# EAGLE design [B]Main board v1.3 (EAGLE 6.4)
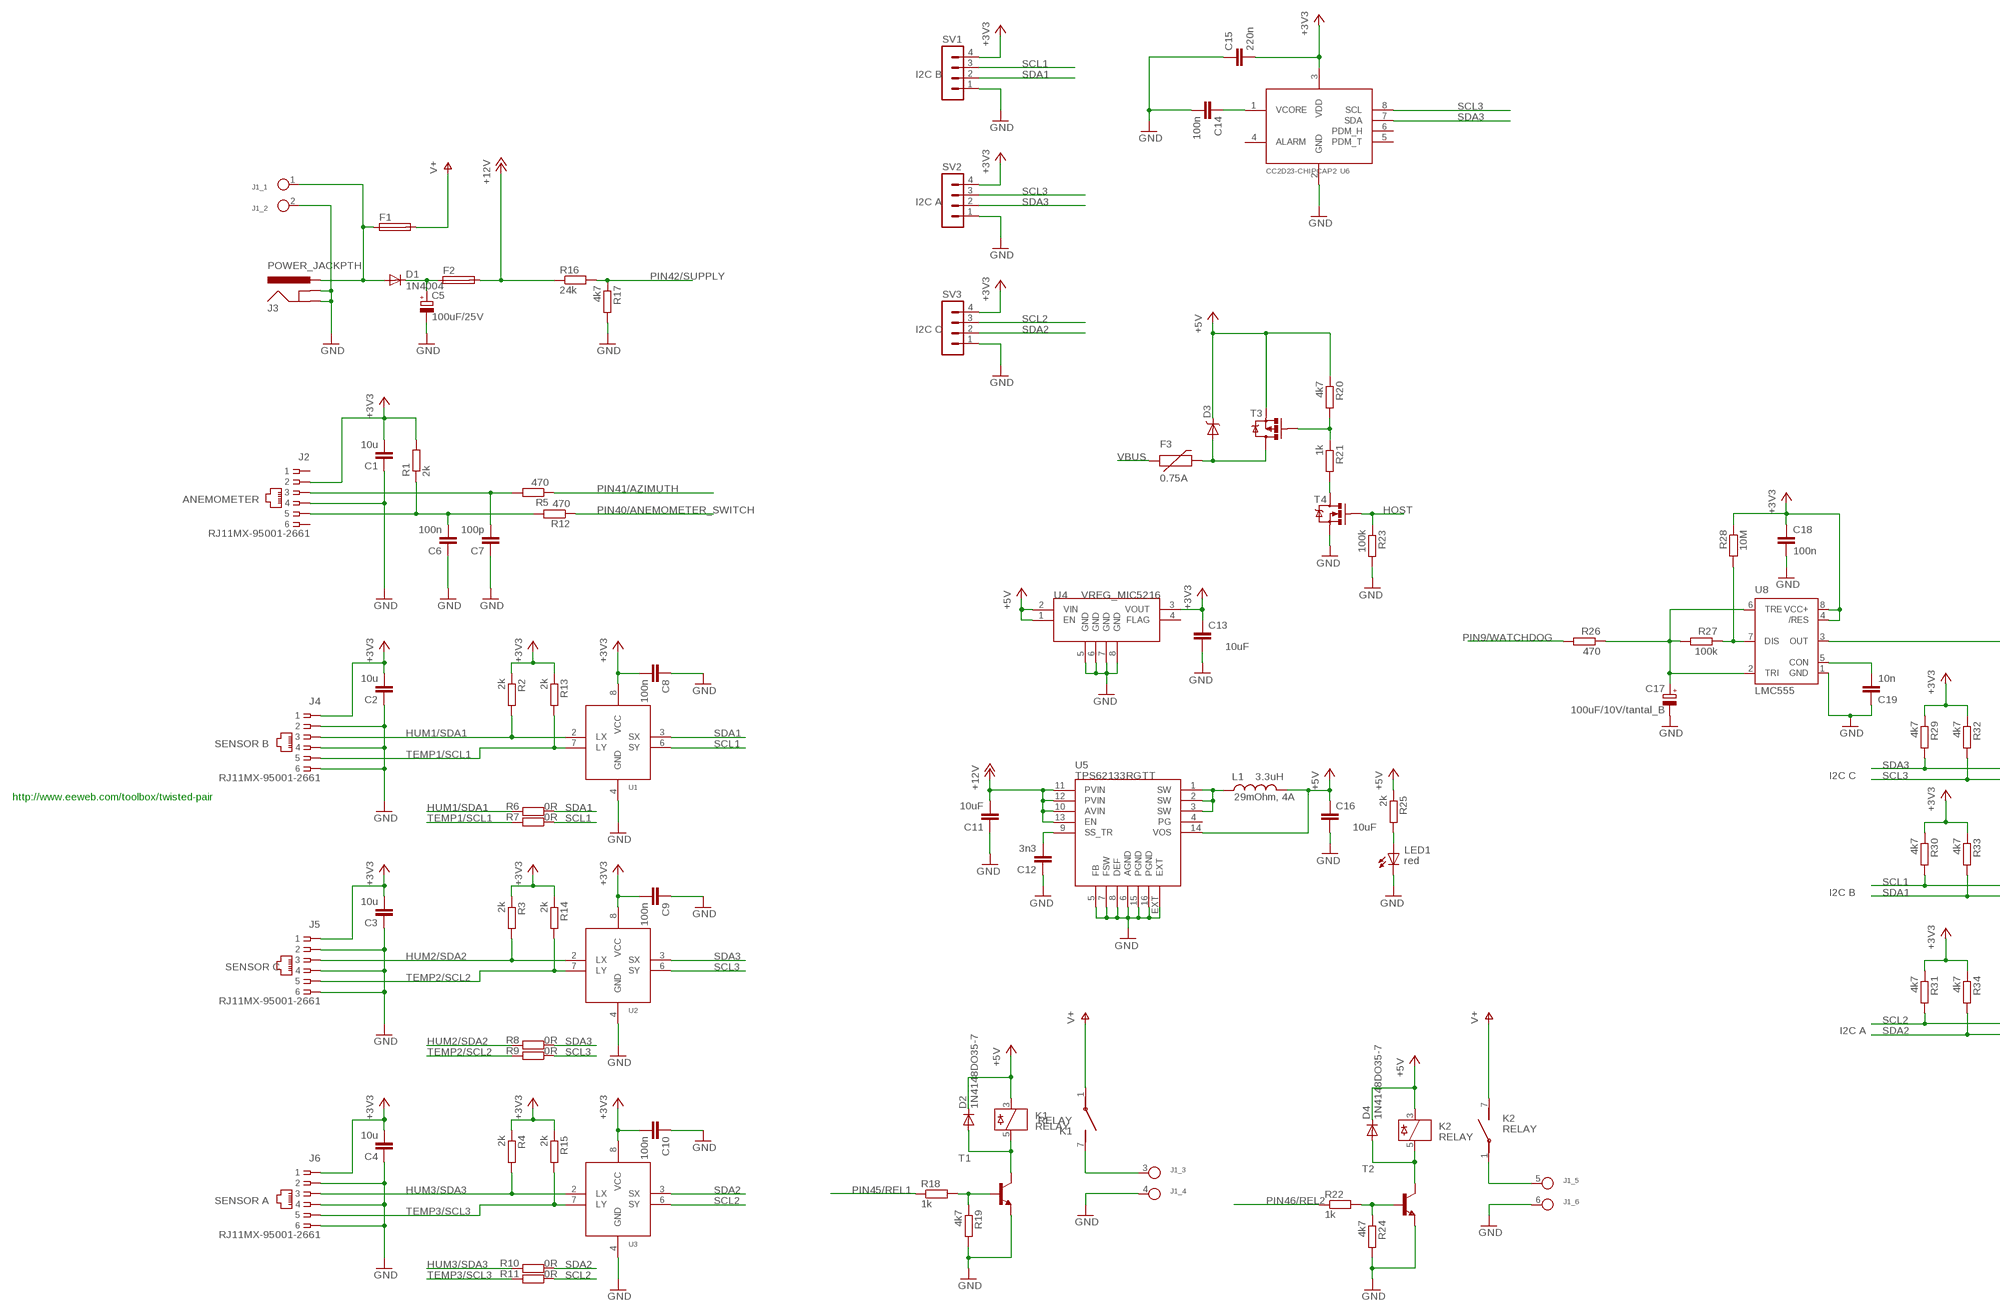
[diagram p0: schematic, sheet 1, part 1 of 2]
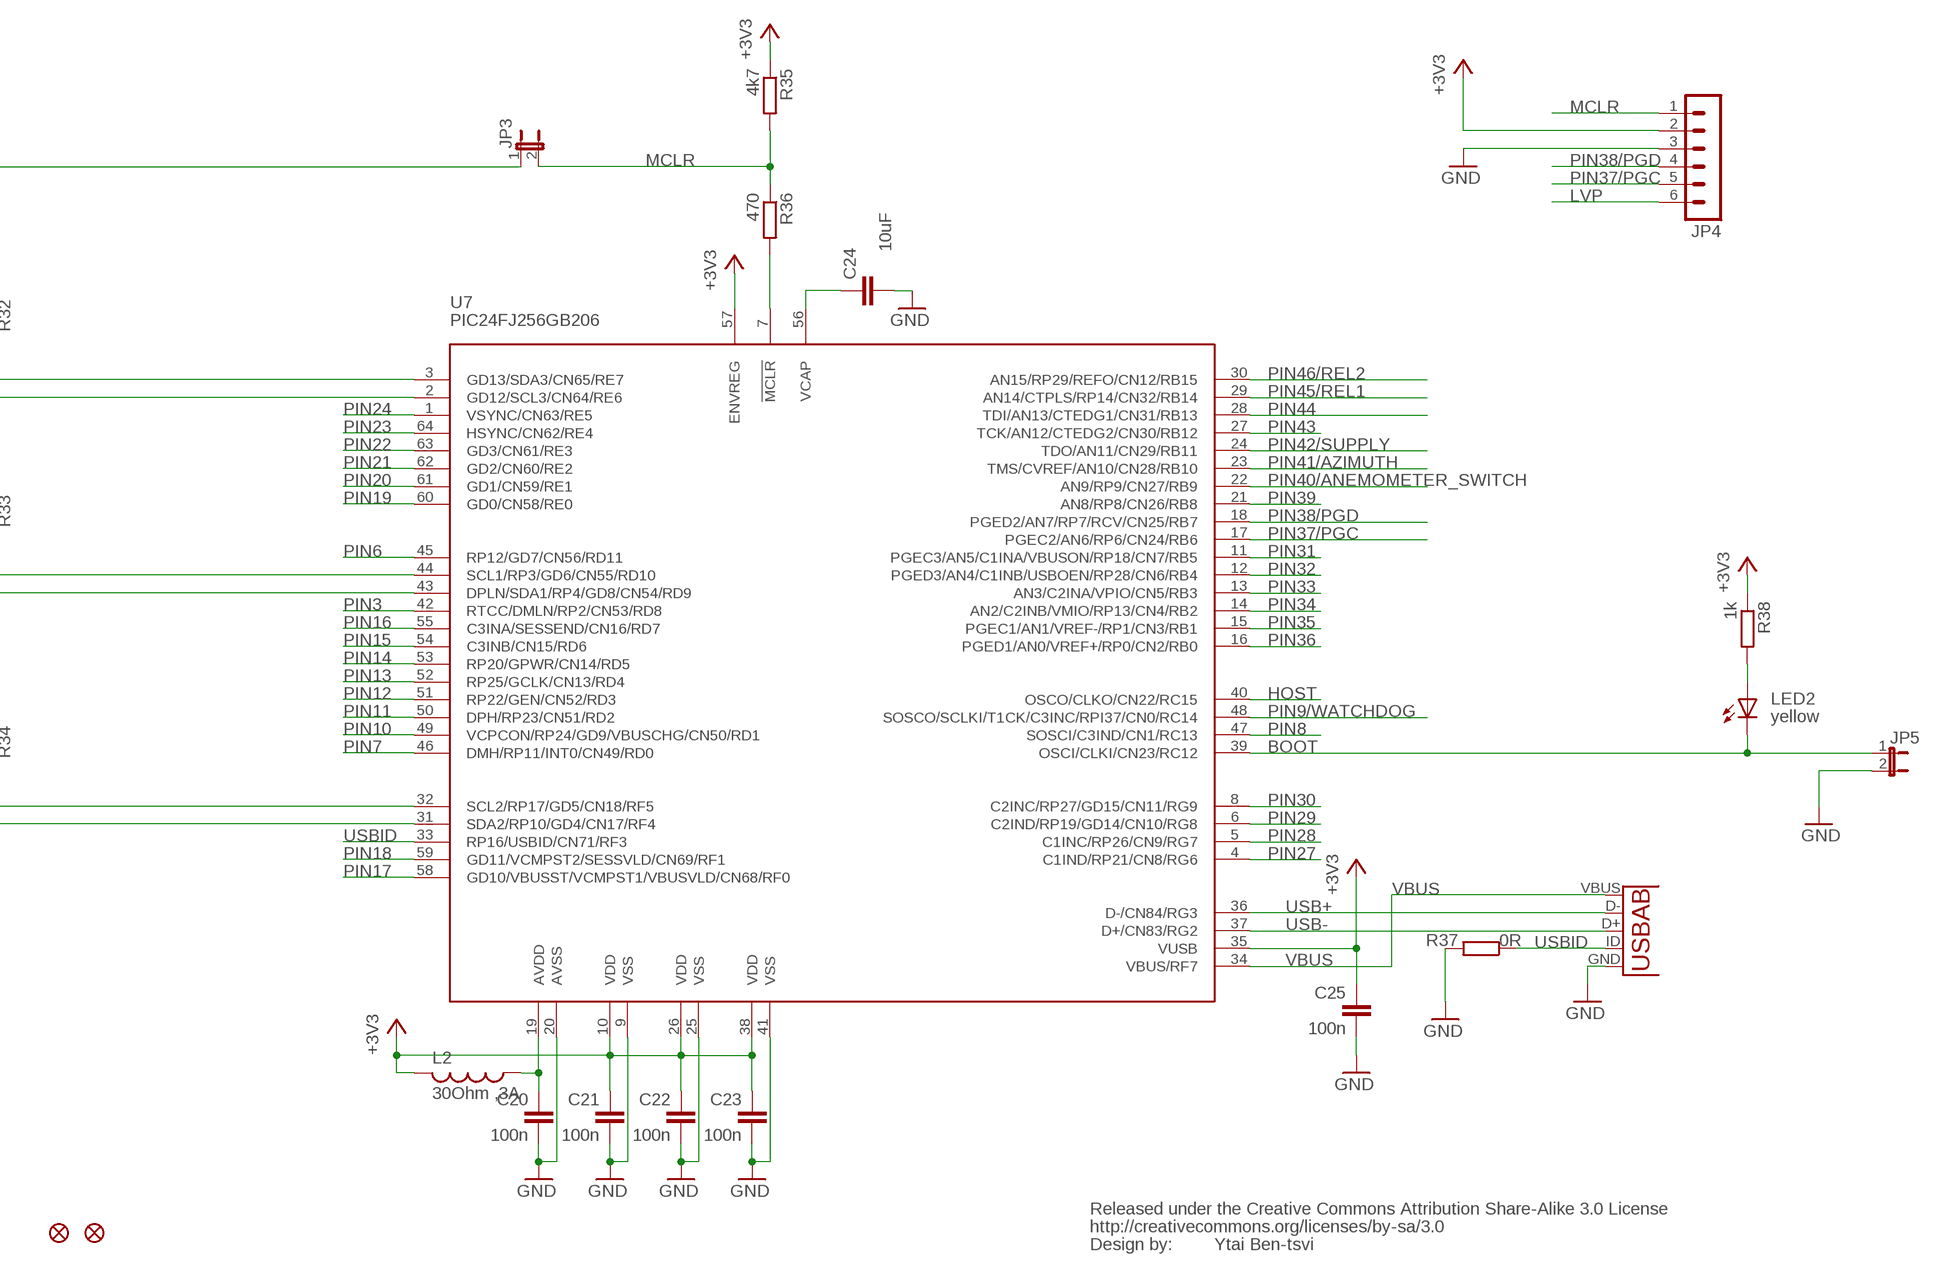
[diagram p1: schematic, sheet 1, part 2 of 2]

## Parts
C1  10u  C-EUC1206  [C1206]
C2  10u  C-EUC1206  [C1206]
C3  10u  C-EUC1206  [C1206]
C4  10u  C-EUC1206  [C1206]
C5  100uF/25V  CPOL-EUE2-5  [E2-5]
C6  100n  C-EUC1206  [C1206]
C7  100p  C-EUC1206  [C1206]
C8  100n  C-EUC1206  [C1206]
C9  100n  C-EUC1206  [C1206]
C10  100n  C-EUC1206  [C1206]
C11  10uF  C-EUC1206  [C1206]
C12  3n3  C-EUC1206  [C1206]
C13  10uF  C-EUC1206  [C1206]
C14  100n  C-EUC1206  [C1206]
C15  220n  C-EUC1206  [C1206]
C16  10uF  C-EUC1206  [C1206]
C17  100uF/10V/tantal_B  CPOL-EUB/3528-21R  [B/3528-21R]
C18  100n  C-EUC1206  [C1206]
C19  10n  C-EUC1206  [C1206]
C20  100n  C-EUC1206  [C1206]
C21  100n  C-EUC1206  [C1206]
C22  100n  C-EUC1206  [C1206]
C23  100n  C-EUC1206  [C1206]
C24  10uF  C-EUC1206  [C1206]
C25  100n  C-EUC1206  [C1206]
D1  1N4004  [DO41-10]
D2  1N4148DO35-7  [DO35-7]
D3  B340A  DIODE-SCHOTTKY_  [SMA-DIODE]
D4  1N4148DO35-7  [DO35-7]
F1  FUSE_HOLDER  [ZHL30]
F2  FUSE_HOLDER  [ZHL30]
F3  PTCSMD  [PTC-1206]
J1  6P_CONN  [MOLEX_39543-0006]
J2  RJ11MX-95001-2661  [MX-95001-2661]
J3  POWER_JACKPTH  [PC-GK2.1]
J4  RJ11MX-95001-2661  [MX-95001-2661]
J5  RJ11MX-95001-2661  [MX-95001-2661]
J6  RJ11MX-95001-2661  [MX-95001-2661]
J7  10104111-0001LF  USB_AB  [USB-AB-MICRO-SMD]
JP1  FIDUCIALUFIDUCIAL  [MICRO-FIDUCIAL]
JP2  FIDUCIALUFIDUCIAL  [MICRO-FIDUCIAL]
JP3  JUMPER-2PTH  [1X02]
JP4  MA06-1  [MA06-1]
JP5  JUMPER-2PTH  [1X02]
K1  RELAY  [JV-5S-KT]
K2  RELAY  [JV-5S-KT]
L1  VLC5045T-3R3N  INDUCTORCR54  [CR54]
L2  30Ohm ,3A  L-US  [R1206]
LED1  LS L29K-G1J2-1-Z  LED1206  [LED-1206]
LED2  LY L29K-J1K2-26-Z  LED1206  [LED-1206]
R1  2k  R-EU_R1206  [R1206]
R2  2k  R-EU_R1206  [R1206]
R3  2k  R-EU_R1206  [R1206]
R4  2k  R-EU_R1206  [R1206]
R5  470  R-EU_R1206  [R1206]
R6  0R  R-EU_R1206  [R1206]
R7  0R  R-EU_R1206  [R1206]
R8  0R  R-EU_R1206  [R1206]
R9  0R  R-EU_R1206  [R1206]
R10  0R  R-EU_R1206  [R1206]
R11  0R  R-EU_R1206  [R1206]
R12  470  R-EU_R1206  [R1206]
R13  2k  R-EU_R1206  [R1206]
R14  2k  R-EU_R1206  [R1206]
R15  2k  R-EU_R1206  [R1206]
R16  24k  R-EU_R1206  [R1206]
R17  4k7  R-EU_R1206  [R1206]
R18  1k  R-EU_R1206  [R1206]
R19  4k7  R-EU_R1206  [R1206]
R20  4k7  R-EU_R1206  [R1206]
R21  1k  R-EU_R1206  [R1206]
R22  1k  R-EU_R1206  [R1206]
R23  100k  R-EU_R1206  [R1206]
R24  4k7  R-EU_R1206  [R1206]
R25  2k  R-EU_R1206  [R1206]
R26  470  R-EU_R1206  [R1206]
R27  100k  R-EU_R1206  [R1206]
R28  10M  R-EU_R1206  [R1206]
R29  4k7  R-EU_R1206  [R1206]
R30  4k7  R-EU_R1206  [R1206]
R31  4k7  R-EU_R1206  [R1206]
R32  4k7  R-EU_R1206  [R1206]
R33  4k7  R-EU_R1206  [R1206]
R34  4k7  R-EU_R1206  [R1206]
R35  4k7  R-EU_R1206  [R1206]
R36  470  R-EU_R1206  [R1206]
R37  0R  R-EU_R1206  [R1206]
R38  1k  R-EU_R1206  [R1206]
SV1  MA04-1  [MA04-1]
SV2  MA04-1  [MA04-1]
SV3  MA04-1  [MA04-1]
T1  BC817-16-NPN-SOT23-BEC  [SOT23-BEC]
T2  BC817-16-NPN-SOT23-BEC  [SOT23-BEC]
T3  IRLML2244  MOSFET-PCHANNELSMD  [SOT23-3]
T4  2N7002PW  MOSFET-NCHANNELSOT323  [SOT323]
U1  P82B715_I2C_BUS_EXTENDER  [SO-08]
U2  P82B715_I2C_BUS_EXTENDER  [SO-08]
U3  P82B715_I2C_BUS_EXTENDER  [SO-08]
U4  VREG_MIC5216  [MSOP8]
U5  TPS62133RGTT  TPS6214X  [QFN16-3X3MM]
U6  CC2D23-CHIPCAP2  [CC2D23-CHIPCAP2]
U7  PIC24FJ256GB206  PIC24FXXXDAX06  [PIC24FXXX_TQFP64]
U8  LMC555  NE555D  [SO08]
U$1  CREATIVE_COMMONS  [CREATIVE_COMMONS]

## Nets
+3V3: C1.2 C2.2 C3.2 C4.2 C8.2 C9.2 C10.2 C13.2 C15.2 C18.1 C21.1 C22.1 C23.1 C25.1 J2.2 J4.1 J5.1 J6.1 JP4.2 L2.2 R1.2 R2.1 R3.1 R4.1 R13.1 R14.1 R15.1 R28.1 R29.1 R30.1 R31.1 R32.1 R33.1 R34.1 R35.1 R38.1 SV1.4 SV2.4 SV3.4 U1.8(VCC) U2.8(VCC) U3.8(VCC) U4.3(VOUT) U6.3(VDD) U7.10(VDD) U7.26(VDD) U7.35(VUSB) U7.38(VDD) U7.57(ENVREG) U8.4(/RES) U8.8(VCC+)
+5V [VCC]: C16.2 D2.C D3.C D4.C K1.3 K2.3 L1.P$2 R20.1 R25.1 T3.2(S) U4.1(EN) U4.2(VIN) U5.14(VOS)
+12V: C11.2 F2.2 R16.1 U5.10(AVIN) U5.11(PVIN) U5.12(PVIN) U5.13(EN)
BOOT: JP5.1 LED2.C U7.39(OSCI/CLKI/CN23/RC12)
GND [VCC]: C1.1 C2.1 C3.1 C4.1 C5.- C6.1 C7.1 C8.1 C9.1 C10.1 C11.1 C12.1 C13.1 C14.2 C15.1 C16.1 C17.- C18.2 C19.1 C20.2 C21.2 C22.2 C23.2 C24.1 C25.2 J1.2 J1.4 J1.6 J2.4 J3.GND J3.GNDBREAK J4.2 J4.4 J4.6 J5.2 J5.4 J5.6 J6.2 J6.4 J6.6 J7.GND JP4.3 JP5.2 LED1.C R17.2 R19.2 R23.2 R24.2 R37.2 SV1.1 SV2.1 SV3.1 T1.E T2.E T4.2(S) U1.4(GND) U2.4(GND) U3.4(GND) U4.5(GND) U4.6(GND) U4.7(GND) U4.8(GND) U5.5(FB) U5.6(AGND) U5.7(FSW) U5.8(DEF) U5.15(PGND) U5.16(PGND) U5.EXT U6.2(GND) U7.9(VSS) U7.20(AVSS) U7.25(VSS) U7.41(VSS) U8.1(GND)
HOST: R23.1 T4.1(G) U7.40(OSCO/CLKO/CN22/RC15)
HUM1/SDA1: J4.3 R2.2 R6.2 U1.2(LX)
HUM2/SDA2: J5.3 R3.2 R8.2 U2.2(LX)
HUM3/SDA3: J6.3 R4.2 R10.2 U3.2(LX)
LVP: JP4.6
MCLR: JP3.2 JP4.1 R35.2 R36.1
N$1: D1.A F1.1 J1.1 J3.PWR
N$2: C6.2 J2.5 R1.1 R12.2
N$3: C5.+ D1.C F2.1
N$4: C7.2 J2.3 R5.2
N$6: C14.1 U6.1(VCORE)
N$9: R36.2 U7.7(!MCLR)
N$10: JP3.1 U8.3(OUT)
N$11: R18.2 R19.1 T1.B
N$12: D2.A K1.5 T1.C
N$13: C19.2 U8.5(CON)
N$16: J1.3 K1.7(2:S)
N$17: C17.+ R26.1 R27.2 U8.2(TRI) U8.6(TRE)
N$19: R27.1 R28.2 U8.7(DIS)
N$20: R22.2 R24.1 T2.B
N$21: D4.A K2.5 T2.C
N$22: C24.2 U7.56(VCAP)
N$23: J1.5 K2.1(2:P)
N$24: LED2.A R38.2
N$25: LED1.A R25.2
N$26: D3.A F3.2 T3.3(D)
N$27: C12.2 U5.9(SS_TR)
N$28: L1.P$1 U5.1(SW) U5.2(SW) U5.3(SW)
N$29: C20.1 L2.1 U7.19(AVDD)
N$30: R20.2 R21.1 T3.1(G)
N$31: R21.2 T4.3(D)
PIN3: U7.42(RTCC/DMLN/RP2/CN53/RD8)
PIN6: U7.45(RP12/GD7/CN56/RD11)
PIN7: U7.46(DMH/RP11/INT0/CN49/RD0)
PIN8: U7.47(SOSCI/C3IND/CN1/RC13)
PIN9/WATCHDOG: R26.2 U7.48(SOSCO/SCLKI/T1CK/C3INC/RPI37/CN0/RC14)
PIN10: U7.49(VCPCON/RP24/GD9/VBUSCHG/CN50/RD1)
PIN11: U7.50(DPH/RP23/CN51/RD2)
PIN12: U7.51(RP22/GEN/CN52/RD3)
PIN13: U7.52(RP25/GCLK/CN13/RD4)
PIN14: U7.53(RP20/GPWR/CN14/RD5)
PIN15: U7.54(C3INB/CN15/RD6)
PIN16: U7.55(C3INA/SESSEND/CN16/RD7)
PIN17: U7.58(GD10/VBUSST/VCMPST1/VBUSVLD/CN68/RF0)
PIN18: U7.59(GD11/VCMPST2/SESSVLD/CN69/RF1)
PIN19: U7.60(GD0/CN58/RE0)
PIN20: U7.61(GD1/CN59/RE1)
PIN21: U7.62(GD2/CN60/RE2)
PIN22: U7.63(GD3/CN61/RE3)
PIN23: U7.64(HSYNC/CN62/RE4)
PIN24: U7.1(VSYNC/CN63/RE5)
PIN27: U7.4(C1IND/RP21/CN8/RG6)
PIN28: U7.5(C1INC/RP26/CN9/RG7)
PIN29: U7.6(C2IND/RP19/GD14/CN10/RG8)
PIN30: U7.8(C2INC/RP27/GD15/CN11/RG9)
PIN31: U7.11(PGEC3/AN5/C1INA/VBUSON/RP18/CN7/RB5)
PIN32: U7.12(PGED3/AN4/C1INB/USBOEN/RP28/CN6/RB4)
PIN33: U7.13(AN3/C2INA/VPIO/CN5/RB3)
PIN34: U7.14(AN2/C2INB/VMIO/RP13/CN4/RB2)
PIN35: U7.15(PGEC1/AN1/VREF-/RP1/CN3/RB1)
PIN36: U7.16(PGED1/AN0/VREF+/RP0/CN2/RB0)
PIN37/PGC: JP4.5 U7.17(PGEC2/AN6/RP6/CN24/RB6)
PIN38/PGD: JP4.4 U7.18(PGED2/AN7/RP7/RCV/CN25/RB7)
PIN39: U7.21(AN8/RP8/CN26/RB8)
PIN40/ANEMOMETER_SWITCH: R12.1 U7.22(AN9/RP9/CN27/RB9)
PIN41/AZIMUTH: R5.1 U7.23(TMS/CVREF/AN10/CN28/RB10)
PIN42/SUPPLY: R16.2 R17.1 U7.24(TDO/AN11/CN29/RB11)
PIN43: U7.27(TCK/AN12/CTEDG2/CN30/RB12)
PIN44: U7.28(TDI/AN13/CTEDG1/CN31/RB13)
PIN45/REL1: R18.1 U7.29(AN14/CTPLS/RP14/CN32/RB14)
PIN46/REL2: R22.1 U7.30(AN15/RP29/REFO/CN12/RB15)
SCL1: R7.1 R30.2 SV1.3 U1.6(SY) U7.44(SCL1/RP3/GD6/CN55/RD10)
SCL2: R11.1 R31.2 SV3.3 U3.6(SY) U7.32(SCL2/RP17/GD5/CN18/RF5)
SCL3: R9.1 R32.2 SV2.3 U2.6(SY) U6.8(SCL) U7.2(GD12/SCL3/CN64/RE6)
SDA1: R6.1 R33.2 SV1.2 U1.3(SX) U7.43(DPLN/SDA1/RP4/GD8/CN54/RD9)
SDA2: R10.1 R34.2 SV3.2 U3.3(SX) U7.31(SDA2/RP10/GD4/CN17/RF4)
SDA3: R8.1 R29.2 SV2.2 U2.3(SX) U6.7(SDA) U7.3(GD13/SDA3/CN65/RE7)
TEMP1/SCL1: J4.5 R7.2 R13.2 U1.7(LY)
TEMP2/SCL2: J5.5 R9.2 R14.2 U2.7(LY)
TEMP3/SCL3: J6.5 R11.2 R15.2 U3.7(LY)
USB+: J7.D- U7.36(D-/CN84/RG3)
USB-: J7.D+ U7.37(D+/CN83/RG2)
USBID: J7.ID(USBID) R37.1 U7.33(RP16/USBID/CN71/RF3)
V+: F1.2 K1.1(2:P) K2.7(2:S)
VBUS: F3.1 J7.VBUS U7.34(VBUS/RF7)
Unconnected: J2.1 J2.6 U4.4(FLAG) U5.4(PG) U6.4(ALARM) U6.5(PDM_T) U6.6(PDM_H)

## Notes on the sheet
- I2C B
- I2C A
- I2C C
- 0.75A
- ANEMOMETER
- SENSOR B
- I2C C
- http://www.eeweb.com/toolbox/twisted-pair | 29mOhm, 4A
- red
- I2C B
- SENSOR C
- yellow
- I2C A
- SENSOR A
- Ytai Ben-tsvi

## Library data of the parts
C1-C4 C6-C16 C18-C25 = rcl:C-EU: CAPACITOR, European symbol
C5 = Thomas Egnal Library:CPOL-EU: POLARIZED CAPACITOR, European symbol
C17 = rcl:CPOL-EU: POLARIZED CAPACITOR, European symbol
D1 = diode:1N4004: DIODE
D2 D4 = diode:1N4148: DIODE
D3 = SparkFun-DiscreteSemi:DIODE-SCHOTTKY: Commonly MBRA140.; PART#: B340A
F1 F2 = Thomas Egnal Library:FUSE_HOLDER: http://www.tme.eu/pl/details/zhl30/bezpieczniki-gniazda-pcb/#t735977d29e6b3d766657895563ce61ae
F3 = SparkFun-PowerIC:PTC: Resettable Fuse PTC; PART#: 0ZCA0075FF2G
J1 = Thomas Egnal Library:6P_CONN
J2 J4-J6 = Thomas Egnal Library:RJ11: CORCOM Modular RJ Jacks No Shield Source: https://www.elfa.se/elfa3~se_sv/elfa/init.do?item=42-696-27&toc=0&q=42-696-27
J3 = Thomas Egnal Library:POWER_JACK: Power Jack This is the standard 5.5mm barrel jack for power. The PTH is the most common, proven, reliable, footprint. All others are experimental. The Slot footprint only works if the mill layer is transmitted to the PCB fab house so be warned. Spark Fun Electronics SKU : PRT-00119. Mating wall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
J7 = SparkFun-Connectors:USB_AB: This is a USB AB connector that is compatible with USB OTG. i.e. this connector can serve as a host or device
JP1 JP2 = SparkFun:FIDUCIAL: Fiducial Alignment Points
JP3 JP5 = SparkFun:JUMPER-2: Jumper
JP4 = con-lstb:MA06-1: PIN HEADER; OC_FARNELL: unknown; OC_NEWARK: unknown
K1 K2 = Thomas Egnal Library:RELAY: JV-5S-KT http://www.tme.eu/pl/details/jv-5s-kt/przekazniki-elektromagn-miniaturowe/fujitsu-takamisawa/#
L1 = SparkFun-Passives:INDUCTOR: Inductors; AM: 3.3uH
L2 = rcl:L-US: INDUCTOR, American symbol
LED1 LED2 = SparkFun:LED: LEDs
R1-R38 = rcl:R-EU_: RESISTOR, European symbol
SV1-SV3 = con-lstb:MA04-1: PIN HEADER; OC_FARNELL: unknown; OC_NEWARK: unknown
T1 T2 = transistor:*-NPN-: NPN Transistror BF959 corrected 2008.03.06
T3 = SparkFun-DiscreteSemi:MOSFET-PCHANNEL: Generic PMOSFET
T4 = SparkFun-DiscreteSemi:MOSFET-NCHANNEL: Generic NMOS footprint; PART#: 2N7002PW
U1-U3 = Thomas Egnal Library:P82B715_I2C_BUS_EXTENDER
U4 = SparkFun-PowerIC:VREG_MIC5216: 500mA LDO, MSOP8 for better dissipation
U5 = SparkFun-PowerIC:TPS6214X: 3-17V, 2A Step Down Converter
U6 = Thomas Egnal Library:CC2D23-CHIPCAP2
U7 = SparkFun-DigitalIC:PIC24FXXXDAX06: PIC24FXXXDAX06 PIC24FXXXDA106 / PIC24FXXXDA206
U8 = SparkFun:NE555: General purpose bipolar Timer
U$1 = SparkFun-Aesthetics:CREATIVE_COMMONS: Creative Commons License summary

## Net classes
1 VCC: width 1.27 mm, clearance 0.254 mm

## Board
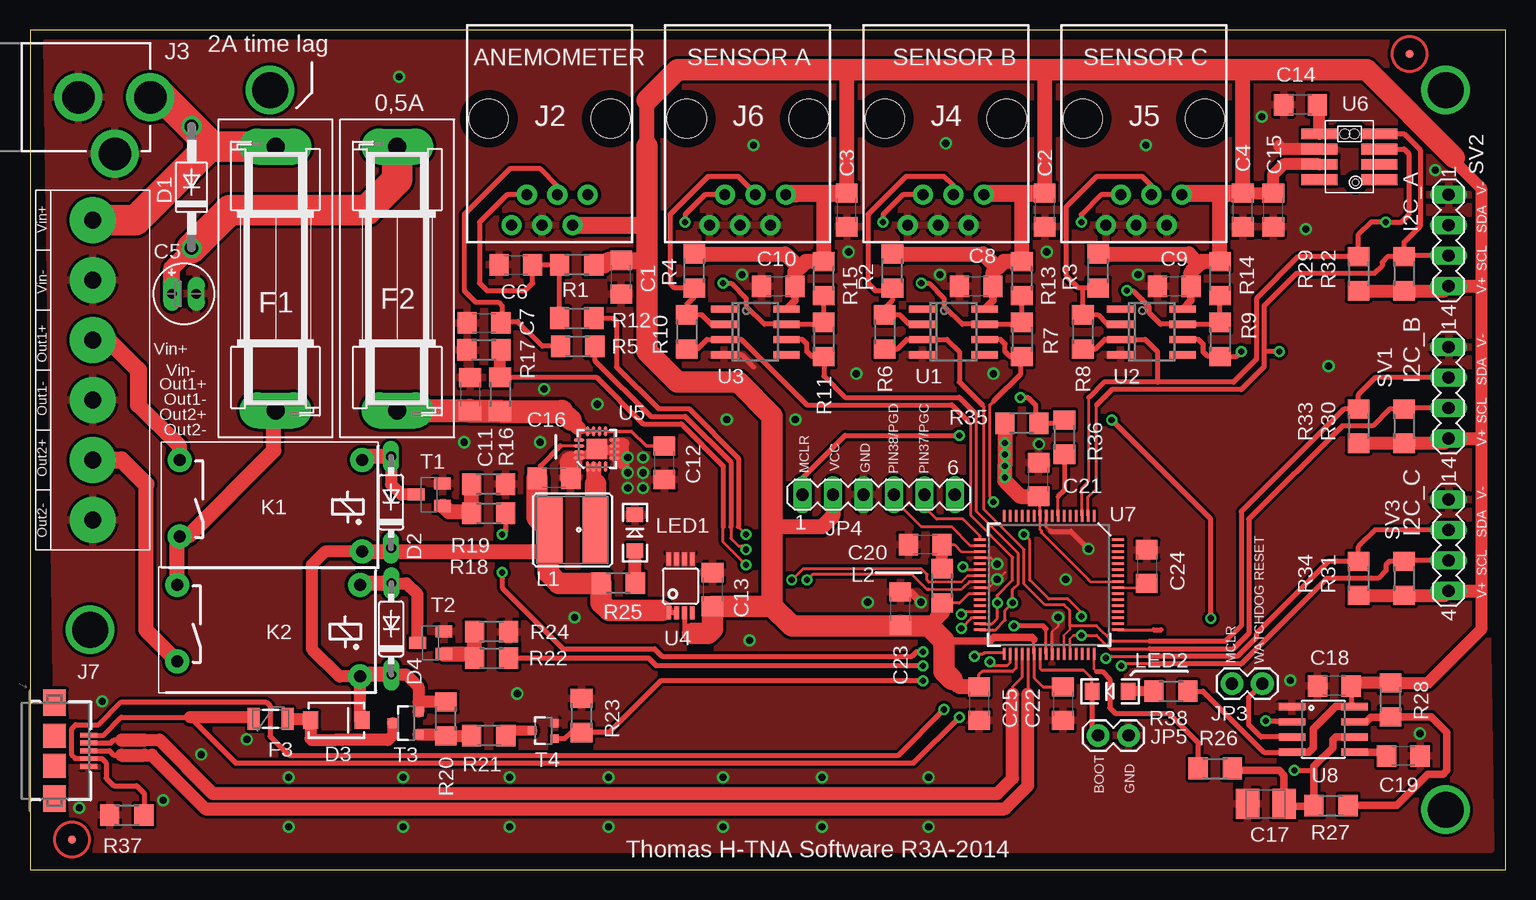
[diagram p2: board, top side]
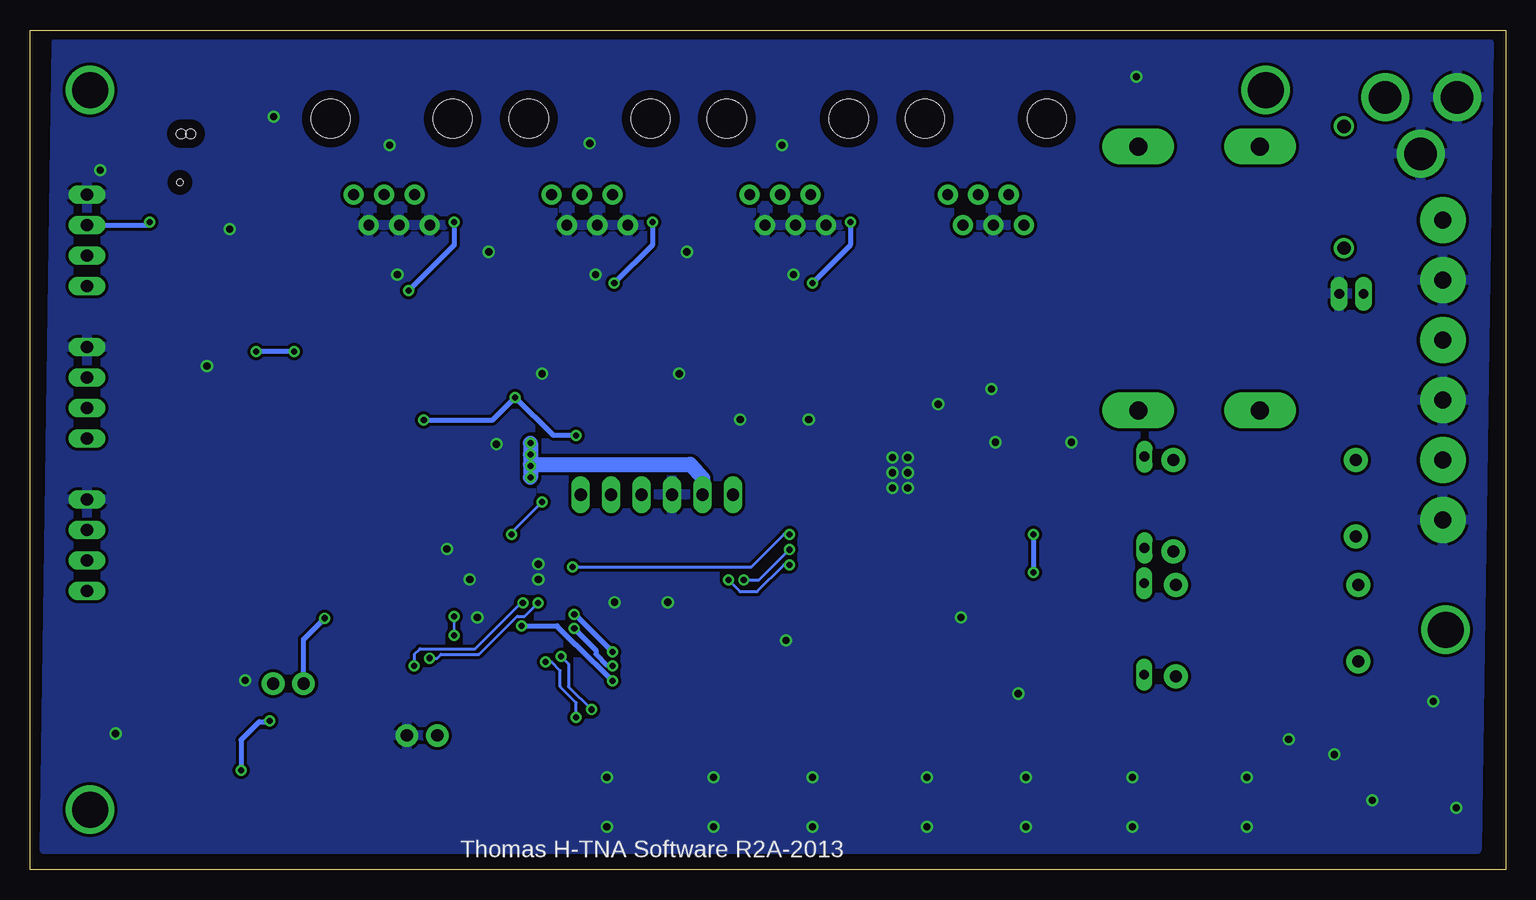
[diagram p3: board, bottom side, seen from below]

Size 123 x 70 mm. Coordinates in mm from the lower left corner, seen from the top.
Outline: 0,0 123,0 123,70 0,70 0,0
Copper layers (1*16): Top 0.035mm / dielectric 1.5mm / Bottom 0.035mm
Design rules "default *": minimum track width 8mil, minimum drill 20mil, track to track 8mil, track to pad 8mil, pad to pad 8mil, via to via 8mil, smd to smd 8mil, copper to edge 30mil, drill to drill 8mil, minimum pad ring 10mil, minimum via ring 8mil, stop-mask expansion 4mil, vias tented up to drill 0mil, thermal gap 10mil

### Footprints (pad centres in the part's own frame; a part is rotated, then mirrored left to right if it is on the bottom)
C1206 = smd 1.6 x 1.8: 1 -1.4,0; 2 1.4,0
E2-5 = drill 0.813 pad 1.397 long: + -1.016,0; - 1.016,0
B/3528-21R = smd 1.95 x 2.5: + 1.525,0; - -1.525,0
DO41-10 = drill 1.118: A 5.08,0; C -5.08,0
DO35-7 = drill 0.813 long: A 3.81,0; C -3.81,0
SMA-DIODE = smd 1.27 x 1.47: A -2.15,0; C 2.15,0
ZHL30 = drill 1.5 pad 3 long: 1 -11,0; 2 11,0
PTC-1206 = smd 1 x 1.8: 1 -1.4,0; 2 1.4,0
MOLEX_39543-0006 = drill 1.4 pad 3.81: 1 -12.5,0; 2 -7.5,0; 3 -2.5,0; 4 2.5,0; 5 7.5,0; 6 12.5,0
MX-95001-2661 = drill 0.9 pad 1.676: 1 -3.175,6.35; 2 -1.905,8.89; 3 -0.635,6.35; 4 0.635,8.89; 5 1.905,6.35; 6 3.175,8.89 | hole 3.251: -5.08,0; 5.08,0
PC-GK2.1 = drill 2.7 pad 4: GND 0,7.7; GNDBREAK 4.7,10.75; PWR 0,13.7
USB-AB-MICRO-SMD = smd 1.4 x 0.4: D+ 2.85,0; D- 2.85,0.65; GND 2.85,-1.3; ID 2.85,-0.65; VBUS 2.85,1.3 | smd 1.9 x 2: P$6 0,1.25; P$7 0,-1.25 | smd 1.9 x 2.2: P$8 0,4; P$9 0,-4
MICRO-FIDUCIAL = smd 0.635 x 0.635: 1 0,0
1X02 = drill 1.016 pad 1.88: 1 0,0; 2 2.54,0
MA06-1 = drill 1.016 long: 1 -6.35,0; 2 -3.81,0; 3 -1.27,0; 4 1.27,0; 5 3.81,0; 6 6.35,0
JV-5S-KT = drill 1 pad 2: 1 16.57,7.54; 3 1.33,8.81; 5 1.33,1.19; 7 16.57,1.19
CR54 = smd 5.5 x 2.15: P$1 0,1.92; P$2 0,-1.92
R1206 = smd 1.6 x 1.803: 1 -1.422,0; 2 1.422,0
LED-1206 = smd 1.2 x 1.4: A -1.5,0; C 1.5,0
MA04-1 = drill 1.016 long: 1 -3.81,0; 2 -1.27,0; 3 1.27,0; 4 3.81,0
SOT23-BEC = smd 1 x 1.4: B -0.95,-1.1; C 0,1.1; E 0.95,-1.1
SOT23-3 = smd 0.8 x 0.9: 1 -0.95,-1; 2 0.95,-1; 3 0,1.1
SOT323 = smd 0.7 x 0.7: 1 -0.65,-0.925; 2 0.65,-0.925; 3 0,0.925
SO-08 = smd 0.6 x 2.2: 1 -1.905,-2.6; 2 -0.635,-2.6; 3 0.635,-2.6; 4 1.905,-2.6; 5 1.905,2.6; 6 0.635,2.6; 7 -0.635,2.6; 8 -1.905,2.6
MSOP8 = smd 0.4 x 1.1: 1 -0.975,-2.25; 2 -0.325,-2.25; 3 0.325,-2.25; 4 0.975,-2.25; 5 0.975,2.25; 6 0.325,2.25; 7 -0.325,2.25; 8 -0.975,2.25
QFN16-3X3MM = smd 0.85 x 0.28: 1 -1.475,0.75; 2 -1.475,0.25; 3 -1.475,-0.25; 4 -1.475,-0.75; 9 1.475,-0.75; 10 1.475,-0.25; 11 1.475,0.25; 12 1.475,0.75 | smd 0.28 x 0.85: 5 -0.75,-1.475; 6 -0.25,-1.475; 7 0.25,-1.475; 8 0.75,-1.475; 13 0.75,1.475; 14 0.25,1.475; 15 -0.25,1.475; 16 -0.75,1.475 | smd 1.68 x 1.68: EXT 0,0
CC2D23-CHIPCAP2 = smd 3 x 0.9: 1 -2.5,1.905; 2 -2.5,0.635; 3 -2.5,-0.635; 4 -2.5,-1.905; 5 2.5,-1.905; 6 2.5,-0.635; 7 2.5,0.635; 8 2.5,1.905 | hole 0.8: -0.4,1.905; 0.4,1.905 | hole 0.5: 0.5,-2.15
PIC24FXXX_TQFP64 = smd 0.22 x 1: 1 -3.75,-5.75; 2 -3.25,-5.75; 3 -2.75,-5.75; 4 -2.25,-5.75; 5 -1.75,-5.75; 6 -1.25,-5.75; 7 -0.75,-5.75; 8 -0.25,-5.75; 9 0.25,-5.75; 10 0.75,-5.75; 11 1.25,-5.75; 12 1.75,-5.75; 13 2.25,-5.75; 14 2.75,-5.75; 15 3.25,-5.75; 16 3.75,-5.75; 33 3.75,5.75; 34 3.25,5.75; 35 2.75,5.75; 36 2.25,5.75; 37 1.75,5.75; 38 1.25,5.75; 39 0.75,5.75; 40 0.25,5.75; 41 -0.25,5.75; 42 -0.75,5.75; 43 -1.25,5.75; 44 -1.75,5.75; 45 -2.25,5.75; 46 -2.75,5.75; 47 -3.25,5.75; 48 -3.75,5.75 | smd 1 x 0.22: 17 5.75,-3.75; 18 5.75,-3.25; 19 5.75,-2.75; 20 5.75,-2.25; 21 5.75,-1.75; 22 5.75,-1.25; 23 5.75,-0.75; 24 5.75,-0.25; 25 5.75,0.25; 26 5.75,0.75; 27 5.75,1.25; 28 5.75,1.75; 29 5.75,2.25; 30 5.75,2.75; 31 5.75,3.25; 32 5.75,3.75; 49 -5.75,3.75; 50 -5.75,3.25; 51 -5.75,2.75; 52 -5.75,2.25; 53 -5.75,1.75; 54 -5.75,1.25; 55 -5.75,0.75; 56 -5.75,0.25; 57 -5.75,-0.25; 58 -5.75,-0.75; 59 -5.75,-1.25; 60 -5.75,-1.75; 61 -5.75,-2.25; 62 -5.75,-2.75; 63 -5.75,-3.25; 64 -5.75,-3.75
SO08 = smd 0.61 x 2.21: 1 -1.905,-2.616; 2 -0.635,-2.616; 3 0.635,-2.616; 4 1.905,-2.616; 5 1.905,2.616; 6 0.635,2.616; 7 -0.635,2.616; 8 -1.905,2.616

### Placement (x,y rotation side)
C1  49.27,49.39 90 top
C2  84.59,54.99 90 top
C3  68.08,54.99 90 top
C4  101.11,54.99 90 top
C5  12.84,48.01 0 top
C6  40.5,50.42 0 top
C7  37.84,45.58 0 top
C8  78.88,48.64 0 top
C9  95.39,48.64 0 top
C10  62.37,48.64 0 top
C11  36.69,39.62 270 top
C12  52.88,33.91 90 top
C13  56.9,23.36 270 top
C14  105.91,63.76 180 top
C15  103.64,54.99 90 top
C16  43.67,32.64 180 top
C17  103.01,5.46 0 top
C18  108.72,15.3 180 top
C19  114.48,9.46 180 top
C20  74.63,27.08 180 top
C21  84.08,32.52 90 top
C22  86.11,13.83 270 top
C23  72.55,21.75 90 top
C24  93.09,25.26 270 top
C25  79.12,13.83 270 top
D1  13.47,56.9 90 top
D2  30.1,30.62 90 top
D3  25.54,12.45 0 top
D4  30.12,20.07 90 top
F1  20.46,49.27 270 top
F2  30.62,49.27 270 top
F3  20.07,12.56 0 top
J1  5.22,41.66 270 top
J2  43.32,62.61 180 top
J3  -3.67,64.38 270 top
J4  76.34,62.61 180 top
J5  92.85,62.61 180 top
J6  59.83,62.61 180 top
J7  2.04,9.9 0 top
JP1  3.5,2.5 0 top
JP2  115,68 0 top
JP3  102.73,15.49 180 top
JP4  70.74,31.25 0 top
JP5  89.04,11.18 0 top
K1  29.04,35.32 180 top
K2  28.83,24.91 180 top
L1  45.23,28.32 270 top
L2  76.04,23.65 270 top
LED1  50.42,28.08 90 top
LED2  90.03,14.86 180 top
R1  45.58,50.42 0 top
R2  71.89,49.91 270 top
R3  89.04,49.91 270 top
R4  55.38,49.91 270 top
R5  45.66,43.64 180 top
R6  71.26,44.83 90 top
R7  82.69,44.2 90 top
R8  87.77,44.83 90 top
R9  99.2,44.2 90 top
R10  54.75,44.83 90 top
R11  66.18,44.2 90 top
R12  45.58,45.98 180 top
R13  82.69,49.27 270 top
R14  99.2,49.27 270 top
R15  66.18,49.27 270 top
R16  39.19,39.62 90 top
R17  37.85,43.32 180 top
R18  38.23,29.7 180 top
R19  38.23,32.13 0 top
R20  34.67,12.56 270 top
R21  38.24,11.18 0 top
R22  38.48,17.64 180 top
R23  45.98,12.84 90 top
R24  38.48,19.82 0 top
R25  49.03,23.88 0 top
R26  98.81,8.43 180 top
R27  108.44,5.33 180 top
R28  113.41,14.15 270 top
R29  110.75,49.67 90 top
R30  114.56,36.97 90 top
R31  114.56,24.27 90 top
R32  114.56,49.67 90 top
R33  110.75,36.97 90 top
R34  110.75,24.27 90 top
R35  82.69,37.21 0 top
R36  86.23,36.05 270 top
R37  8.08,4.54 180 top
R38  95.11,14.86 180 top
SV1  118.25,39.75 270 top
SV2  118.25,52.45 270 top
SV3  118.25,27.05 270 top
T1  33.27,31.25 90 top
T2  33.4,18.91 90 top
T3  31.37,12.21 90 top
T4  42.8,11.57 90 top
U1  76.97,44.83 270 top
U2  93.48,44.83 270 top
U3  60.47,44.83 270 top
U4  54.23,23.64 0 top
U5  47.24,35.06 90 top
U6  110,59.44 0 top
U7  84.95,23.75 180 top
U8  107.81,11.69 270 top
U$1  not placed on the board

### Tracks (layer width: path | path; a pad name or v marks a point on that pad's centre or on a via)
+3V3  (via drill 0.51)
  Top 0.203: U7.10 84.2,28.35 84.3,28.26 | U7.57 88.39,24 88.27,24.13
  Top 0.254: U7.35 82.2,16.8 81.92,16.51 79.38,16.51 79.12,16.25 C25.1 | 83.7,19.17 U7.38 83.7,15.99 84.45,15.24 86.09,15.24 C22.1 | U7.10 84.2,31.64 C21.1 | U7.26 78.25,23 77.47,22.23 L2.2 | 84.3,28.26 84.3,28.1 88.27,24.13
  Top 0.406: U4.3 54.55,19.74 54.61,19.68 54.61,20.32 55.24,20.32 55.24,19.68 | C18.1 110.12,13.89 U8.8 | U8.4 102.87,9.78 97.79,14.86 R38.1 | 81.28,33.78 v81.28,33.66 v81.28,32.7
  Top 0.61: U8.8 108.84,13.59 107,11.75 107,10.16 106.62,9.78 U8.4 | C8.2 80.28,47.44 U1.8 | C10.2 63.77,47.44 U3.8 | C9.2 96.79,47.44 U2.8 | 76.2,19.05 80.01,19.05 80.3,19.34 83.53,19.34 83.7,19.17
  Top 1.016: C4.2 C15.2 103.64,57.92 104.52,58.8 U6.3 | 118.75,59.37 118.75,59.05 120.97,56.83 120.97,48.9 120.97,36.2 120.97,23.5 120.97,20 116.53,15.57 R28.1 110.39,15.57 C18.1 | 61.59,26.67 61.59,23.13 61.87,22.86
  Top 1.067: 120.97,48.9 120.71,48.64 SV2.4 117.86,48.25 R32.1 R29.1 | R33.1 R30.1 117.86,35.55 SV1.4 120.71,35.94 120.97,36.2 | 120.97,23.5 120.71,23.24 SV3.4 117.86,22.85 R31.1 R34.1
  Top 1.27: 51.44,60.33 51.44,64.14 | C2.2 84.59,66.53 84.45,66.67 | J6.1 63.88,56.26 | C3.2 68.08,66.53 67.94,66.67 | C4.2 101.11,66.53 100.97,66.67 | 66.04,56.39 66.18,56.25 R15.1 64.67,50.7 64.14,50.16 | C10.2 63.77,49.8 64.14,50.16 | R4.1 62.97,51.33 64.14,50.16 | 82.55,56.39 82.69,56.25 R13.1 81.18,50.7 80.64,50.16 | 80.64,50.16 80.28,49.8 C8.2 | R2.1 79.48,51.33 80.64,50.16 | 99.06,56.39 99.2,56.25 R14.1 97.69,50.7 97.47,50.48 | C9.2 96.79,49.8 97.47,50.48 | R3.1 96.62,51.33 97.47,50.48 | C25.1 77.48,15.23 76.83,15.88 | L2.2 76.04,21.43 74.93,20.32 | JP4.2 66.93,29.46 66.04,28.57 61.87,28.57 | R35.1 81.27,33.64 | 81.27,33.64 81.27,32.4 82.55,31.11 84.06,31.11 C21.1 | 81.27,33.64 81.28,33.78
  Top 1.422: J2.2 51.05,53.72 51.44,53.34 | 51.44,50.8 51.42,50.79 C1.2 48.26,50.8 47.88,50.42 R1.2 | J6.1 63.01,56.39 66.04,56.39 C3.2 | J4.1 79.52,56.39 82.55,56.39 C2.2 | J5.1 96.03,56.39 99.06,56.39 C4.2
  Top 1.778: 61.87,21.95 C13.2 56.9,20.07 56.52,19.68 55.24,19.68 | 51.44,60.33 51.44,53.34 51.44,50.8 51.44,43.18 53.98,40.64 59.05,40.64 61.87,37.83 61.87,28.57 61.87,22.86 61.87,21.95 | 51.44,64.14 53.98,66.67 67.94,66.67 84.45,66.67 100.97,66.67 111.44,66.67 118.75,59.37 | 61.87,21.95 63.5,20.32 72.58,20.32 | 76.83,15.88 76.2,16.51 76.2,19.05 74.93,20.32 72.58,20.32 | 72.58,20.32 C23.1
  Bottom 1.27: 81.28,33.78 67.94,33.78 66.93,32.64 JP4.2 | v81.28,35.56 v81.28,34.61 81.28,33.78 | 81.28,33.78 v81.28,32.7
+5V
  Top 0.254: U5.14 44.2,35.31
  Top 0.305: 43.81,29.75 43.22,29.14
  Top 0.406: 44.2,35.31 42.55,33.66 42.55,32.91 C16.2 | U4.2 53.34,21.39 U4.1 52.91,21.39 52.7,21.59
  Top 1.016: 30.95,26.51 29.8,26.51 24.61,26.51 23.5,25.4 23.5,18.41 25.82,16.09 K2.3 27.5,12.45 D3.C | 43.18,27.94 43.18,29.46 43.22,29.14 L1.P$2 | D4.C 31.37,16.25 32.38,15.24 32.38,13.97 | 32.38,13.97 32.38,13.17 T3.2 | R20.1 32.4,13.98 32.38,13.97
  Top 1.27: K1.3 29.8,26.51 D2.C | D4.C 27.66,16.25 K2.3 | 30.95,26.51 43.02,26.51 43.18,26.67 43.18,28.2 L1.P$2
  Top 1.778: C16.2 42.29,29.34 L1.P$2 | 43.18,26.67 43.18,24.77 44.07,23.88 R25.1 47.61,22.24 48.26,21.59 52.7,21.59
+12V
  Top 0.254: U5.13 45.77,35.97 | U5.10 U5.11
  Top 0.305: 45.77,36.78 45.72,36.83
  Top 0.406: U5.11 U5.12 46.01,36.54 45.77,36.78 | 45.77,35.97 45.77,36.78 | 45.77,36.78 45.72,36.83
  Top 1.27: 45.72,36.83 45.09,37.47
  Top 1.778: 44.35,38.2 45.09,37.47
  Top 1.93: F2.2 36.64,38.27 C11.2 39.17,38.23 R16.1 44.35,38.2
BOOT
  Top 0.254: LED2.C 88.53,15.93 87.82,16.64 84.33,16.64 84.2,16.77 U7.39
  Top 0.406: LED2.C 88.53,11.69 JP5.1
GND  (via drill 0.6 pad 0.81)
  Top 0.203: U7.9 84.7,28.58 85.09,28.19 | U7.25 79.93,23.5 v80.63,24.19 80.64,24.18 81.28,24.77 | U7.20 80.09,26 v80.63,25.46 | U7.41 85.2,19.8 85.72,20.32 85.72,21 v85.71,21.02
  Top 0.254: U5.EXT 47.1,34.92 46.99,34.92 46.88,34.81 U5.15 U5.16 45.77,34.37 46,34.59 46.46,34.59 46.46,34.42 46.41,34.37 45.16,34.37 45.11,34.31
  Top 0.305: 45.11,34.31 45.09,34.29 45.09,33.97 45.09,33.66
  Top 0.406: U5.EXT 48.47,35.06 | U3.4 59.31,42.92 60.33,41.91 | 85.09,28.19 86.78,28.19 v88.25,26.73
  Top 0.61: C23.2 73.42,23.15 v74.28,22.29
  Top 0.813: U5.6 48.72,34.47 49.53,33.66 49.53,35.56 48.9,35.56 48.9,34.92 47.38,34.92 U5.EXT
  Top 1.016: U6.2 104.39,60.07 104.14,60.33
  Top 1.778: C16.1 45.08,33.96 45.09,33.97
  other vias: 76.34,60.55 60.31,60.39 30.78,66.1 59.99,19.11 42.84,40.07 47.29,38.8 108.25,41.97 45.38,21.02 93.01,60.39 11.09,5.78 21.57,7.68 21.57,3.56 31.1,3.56 39.99,3.56 48.24,3.56 57.77,3.56 66.02,3.56 74.91,3.56 14.27,9.59 31.1,7.68 39.99,7.68 48.24,7.68 57.77,7.68 66.02,7.68 74.91,7.68 42.53,35.62 36.18,35.62 4.11,5.14 6.01,14.03 59.35,49.59 75.86,49.59 92.37,49.59 86.34,24.19 18.08,10.86 40.62,14.67 51.1,34.35 49.83,34.35 49.83,33.08 49.83,31.81 51.1,33.08 51.1,31.81 63.8,37.53 58.08,37.53 69.83,22.29 117.14,58.32 68.88,41.34 80.31,41.34 68.24,51.5 115.87,11.33 105.07,15.78 102.69,62.77 84.12,35.46 106.34,53.4 84.75,51.5
  pour Top: 120.79,68.96 1.41,68.96 2.41,1.68 121.79,1.68
  pour Bottom: 120.79,68.96 1.41,68.96 2.41,1.68 121.79,1.68
HOST  (via drill 0.51)
  Top 0.254: U7.40 84.7,20.07
  Top 0.406: T4.1 44.58,10.92 45.09,11.43 45.96,11.43 R23.1 48.26,11.43 52.55,15.72 v74.45,15.72 | 84.7,20.07 84.45,20.32 v82.01,20.32
  Bottom 0.406: v82.01,20.32 79.06,20.32 79.06,20.26 77.53,18.73 77.47,18.73 v74.45,15.72
HUM1/SDA1
  Top 0.406: J4.3 76.97,57.01 76.2,57.78 73.03,57.78 69.85,54.61 69.85,48.9 70.48,48.26 71.67,48.26 R2.2 71.89,47.45 71.26,46.81 R6.2 72.49,46.25 73.28,45.47 U1.2
HUM2/SDA2
  Top 0.406: J5.3 93.48,57.01 92.71,57.78 88.9,57.78 86.36,55.24 86.36,49.53 87.4,48.49 87.63,48.49 | R3.2 87.63,48.49 | U2.2 89.79,45.47 89,46.25 R8.2 87.77,48.35 87.63,48.49
HUM3/SDA3
  Top 0.406: J6.3 60.47,56.38 59.05,57.78 56.52,57.78 53.34,54.61 53.34,48.9 53.75,48.49 R4.2 55.38,47.77 54.75,47.13 R10.2 55.98,46.25 56.77,45.47 U3.2
MCLR  (via drill 0.51)
  Top 0.406: JP4.1 64.39,32.64 67.94,36.2 v77.47,36.2 | v82.55,39.37 83.19,39.37 83.82,38.73 83.82,37.5 R35.2 85.84,37.21 R36.1 | v98.42,20.95 98.42,29.21 v90.17,37.47
  Bottom 0.406: v77.47,36.2 79.38,36.2 v82.55,39.37 84.45,37.47 v90.17,37.47 | JP3.2 100.19,19.19 v98.42,20.95
N$1
  Top 2.54: J3.PWR 11.07,64.38 D1.A 15.06,60.39 | 15.06,60.39 15.18,60.27 F1.1 | J1.1 8.83,54.16 15.06,60.39
N$2
  Top 0.406: J2.5 39.75,56.26 37.47,53.98 37.47,48.9 38.1,48.26 41.27,48.26 41.91,48.9 C6.2 R1.1 R12.2
N$3
  Top 1.422: C5.+ 11.82,50.16 D1.C
  Top 2.54: D1.C 16.65,54.99 28.08,54.99 30.62,57.53 F2.1
N$4
  Top 0.406: J2.3 43.95,57.01 42.55,58.42 40.01,58.42 36.2,54.61 36.2,48.26 37.15,47.31 39.05,47.31 39.37,46.99 39.37,45.7 | 39.37,45.7 C7.2 | 39.37,45.7 40.66,45.7 42.72,43.64 R5.2
N$5  (via drill 3 pad 4)
  other vias: 20,65
N$6
  Top 1.016: U6.1 107.5,63.56 C14.1
N$7  (via drill 3 pad 4)
  other vias: 5,20
N$8  (via drill 3 pad 4)
  other vias: 118,5
N$9
  Top 0.254: U7.7 85.7,31.09
  Top 0.406: 85.7,31.09 86.23,31.62 R36.2
N$10
  Top 0.406: U8.3 102.61,11.05 101.6,12.06 101.6,14.37 JP3.1
N$11
  Top 1.27: T1.B 34.47,30.3 34.92,29.84 36.66,29.84 R18.2 R19.1
N$12
  Top 1.016: T1.C 30.98,31.25 30.1,32.13 D2.A
  Top 1.27: D2.A 28,34.43 K1.5
N$13
  Top 0.61: U8.5 112.76,9.78 C19.2
N$14  (via drill 3 pad 4)
  other vias: 118,65
N$16
  Top 1.27: K1.7 12.46,35.3 9.03,38.73
  Top 1.422: J1.3 6.53,44.16 9.03,41.66 9.03,38.73
N$17  (via drill 0.51)
  Top 0.203: 100.61,8.26 100.4,8.26 R26.1
  Top 0.406: 103.89,12.32 U8.2 105.13,12.38 v103.03,12.38 | v105.41,8.26 107.02,8.26
  Top 0.61: U8.6 108.84,11.05 108.58,10.79 108.58,10.16 107.02,8.6 107.02,8.26 R27.2 106.94,5.26 104.74,5.26 C17.+ 104.53,7.86 104.14,8.26 100.61,8.26
  Bottom 0.406: v105.41,8.26 105.41,10.79 103.89,12.32 103.09,12.32 v103.03,12.38
N$19
  Top 0.61: U8.7 111.38,12.32 111.76,12.7 113.39,12.7 R28.2 116.81,12.73 118.11,11.43 118.11,8.26 117.79,7.94 116.52,7.94 113.92,5.33 R27.1
N$20
  Top 1.27: T2.B 36.74,17.96 R22.2 R24.1
N$21
  Top 1.016: D4.A 31.37,23.88 32.3,22.95 T2.C
  Top 1.27: K2.5 27.66,23.88 D4.A 30.23,23.99
N$22
  Top 0.203: U7.56 92.73,23.5 C24.2
N$23
  Top 1.27: 9.66,32.13 9.66,19.96 K2.1
  Top 1.422: J1.5 7.64,34.16 9.66,32.13
N$24
  Top 0.813: R38.2 LED2.A
N$25
  Top 1.067: R25.2 50.46,26.54 LED1.A
N$26
  Top 1.016: F3.2 23.39,12.56 D3.A 23.39,10.9 23.5,10.79 25.4,10.79 26.04,10.79 29.84,10.79 30.27,11.22 T3.3
N$27
  Top 0.305: C12.2 51.4,35.31 50.16,36.54 U5.9
N$28
  Top 0.254: U5.1 46.49,32.35 46.58,32.26 47.02,32.26 47.15,32.13 | 47.85,32.41 47.49,32.77 U5.3 U5.2
  Top 0.813: U5.2 46.99,32.28 47.02,32.26
  Top 1.778: L1.P$1 47.15,32.13 47.14,32.13
N$29
  Top 0.203: U7.19 77.64,26.5
  Top 0.254: C20.1 77.06,27.08 77.64,26.5
  Top 1.016: L2.1 C20.1
N$30
  Top 1.016: T3.1 34.55,11.26 R20.2 36.78,11.14 R21.1
N$31
  Top 0.813: T4.3 40.06,11.57 R21.2
PIN9/WATCHDOG
  Top 0.203: U7.48 88.7,16.71 88.9,16.51
  Top 0.406: 88.9,16.51 89.38,16.51 90.01,15.88 90.01,13.49 90.49,13.02 94.93,13.02 97.38,10.57 R26.2
PIN10
  Top 0.254: U7.49 93.67,20
  Top 0.406: 93.67,20 94.3,20
PIN37/PGC
  Top 0.254: U7.17 79.2,27.8 77.79,29.21 75.56,29.21 74.55,30.23 JP4.5
PIN38/PGD
  Top 0.254: U7.18 78.41,27 76.83,28.57 74.3,28.57 72.39,30.48 72.39,30.88 JP4.4
PIN40/ANEMOMETER_SWITCH  (via drill 0.51)
  Top 0.254: U7.22 78.03,25 v77.79,25.24 | 59.05,28.57 v59.69,27.94
  Top 0.406: R12.1 48.64,45.98 48.9,45.72 48.9,41.91 52.39,38.42 54.93,38.42 59.05,34.29 59.05,28.57
  Bottom 0.254: v77.79,25.24 62.87,25.24 60.17,27.94 v59.69,27.94
PIN41/AZIMUTH  (via drill 0.51)
  Top 0.203: 78.16,24.5 77.63,23.97 74.93,23.97
  Top 0.254: v63.5,24.13 64.45,25.08 74.3,25.08 74.77,24.61 74.77,24.13 74.93,23.97 | U7.23 78.16,24.5 | 58.42,28.57 58.42,27.62 59.05,26.99 59.37,26.99 v59.69,26.67
  Top 0.406: R5.1 47.08,42.46 51.75,37.78 54.61,37.78 58.42,33.97 58.42,28.57
  Bottom 0.254: v63.5,24.13 62.23,24.13 v59.69,26.67
PIN42/SUPPLY  (via drill 0.51)
  Top 0.203: 77.79,23.5 77.63,23.34 74.93,23.34
  Top 0.254: v64.77,24.13 65.25,24.61 73.5,24.61 74.77,23.34 74.93,23.34 | U7.24 78.29,24 77.79,23.5 | v59.69,25.4 57.78,27.3 57.78,28.57
  Top 0.406: R16.2 47.22,41.05 51.12,37.15 54.29,37.15 57.78,33.66 57.78,28.57
  Top 1.016: R16.2 39.19,43.24 R17.1
  Bottom 0.254: v64.77,24.13 63.82,23.18 62.39,23.18 60.17,25.4 v59.69,25.4
PIN45/REL1  (via drill 0.51)
  Top 0.254: U7.29 77.86,21.5 v77.63,21.27
  Top 0.406: R18.1 39.65,28.22 v39.37,27.94 | v39.37,24.77 39.37,23.5 44.45,18.41 52.07,18.41 52.7,17.78 73.5,17.78 73.88,18.16 v74.45,18.16
  Bottom 0.406: v39.37,27.94 v39.37,24.77 | v77.63,21.27 77.56,21.27 v74.45,18.16
PIN46/REL2  (via drill 0.51)
  Top 0.254: U7.30 78.47,21 v77.63,20.1
  Top 0.406: v74.45,16.99 52.23,16.99 51.58,17.64 R22.1
  Bottom 0.406: v74.45,16.99 74.83,16.99 75.82,17.97 75.82,18.29 v77.63,20.1
SCL1  (via drill 0.51)
  Top 0.203: U7.44 86.7,19.23 87,19.53 v87.63,19.53
  Top 0.254: 93.34,18.41 90.01,18.41 88.9,19.53 v87.63,19.53 | v87.63,21.11 87.63,21.43 86.52,22.54 84.93,22.54 83.34,24.13 83.34,27.46 v82.87,27.94 | v80.33,30.64 80.33,30.8 80.01,31.11 80.01,38.73 80.33,39.05
  Top 0.406: R7.1 82.32,42.77 | SV1.3 114.64,38.48 R30.2 113.32,38.39 111.92,36.99 109.38,36.99 101.6,29.21 101.6,19.68 100.33,18.41 93.34,18.41 | U1.6 80.9,44.2 81.28,43.81 81.28,43.18 81.69,42.77 82.32,42.77 | 82.32,42.77 82.55,42.55 82.55,41.27 80.33,39.05
  Bottom 0.203: v87.63,19.53 v87.63,21.11
  Bottom 0.254: v82.87,27.94 82.87,28.1 v80.33,30.64
SCL2  (via drill 0.51)
  Top 0.254: U7.32 80.48,20 81.28,20.8 81.28,21.59 v81.92,22.23 81.92,23.34 82.39,23.81 82.39,26.35 78.9,29.84 78.9,37.94 78.74,38.1 | 93.34,17.14 91.12,17.14 v90.96,16.99
  Top 0.406: SV3.3 114.64,25.78 R31.2 113.32,25.69 113.03,25.4 113.03,24.92 112.39,24.29 108.11,24.29 100.97,17.14 93.34,17.14 | 78.74,38.1 77.47,39.37 67.94,39.37 66.18,41.13 R11.1 65.18,42.77 64.77,43.18 64.77,43.81 64.39,44.2 U3.6
  Bottom 0.254: v81.92,22.23 82.07,22.23 85.88,18.41 90.49,18.41 90.96,17.94 v90.96,16.99
SCL3  (via drill 0.51)
  Top 0.254: U7.2 88.2,31.05 88.9,31.75 88.9,38.73
  Top 0.406: U6.8 114.56,61.34 115.89,60.01 115.89,53.66 114.56,52.33 R32.2 | SV2.3 114.64,51.18 R32.2 | R32.2 113.16,51.09 112.71,50.64 112.71,50.32 112.08,49.69 105.57,49.69 102.87,46.99 102.87,43.18 | U2.6 97.41,44.2 97.79,43.81 97.79,43.18 98.2,42.77 R9.1 100.56,42.77 v100.97,43.18 | 102.87,43.18 102.87,41.91 100.97,40.01 90.17,40.01 88.9,38.73 | v104.14,43.18 102.87,43.18
  Bottom 0.406: v100.97,43.18 v104.14,43.18
SDA1
  Top 0.203: U7.43 86.2,19.52 86.68,20 86.68,20.32
  Top 0.254: 93.34,19.05 90.17,19.05 88.9,20.32 86.68,20.32 86.68,21.59 86.2,22.07 84.61,22.07 82.87,23.81 82.87,26.67 79.53,30 79.53,38.58 79.38,38.73
  Top 0.406: R6.1 72.3,43.41 73.09,44.2 U1.3 76.45,44.2 77.47,43.18 77.47,40.64 79.38,38.73 | SV1.2 112.14,41.02 110.75,39.62 R33.2 109.51,38.39 100.97,29.84 100.97,20.32 99.69,19.05 93.34,19.05
SDA2  (via drill 0.51)
  Top 0.254: U7.31 80.19,20.5 80.64,20.95 v80.64,22.23 80.64,22.86 81.92,24.13 81.92,26.04 78.42,29.53 78.42,37.15 78.11,37.47 | v89.69,17.62 90.01,17.62 90.17,17.78 93.34,17.78
  Top 0.406: R10.1 55.63,43.41 56.42,44.2 U3.3 59.31,44.2 64.77,38.73 76.83,38.73 78.11,37.47 | SV3.2 112.14,28.32 110.75,26.93 R34.2 108.24,25.69 102.23,19.68 102.23,19.37 100.65,17.78 93.34,17.78
  Bottom 0.254: v89.69,17.62 89.06,17.62 88.74,17.94 85.57,17.94 82.39,21.11 81.76,21.11 v80.64,22.23
SDA3  (via drill 0.51)
  Top 0.254: U7.3 87.7,31.82 88.27,32.38 88.27,39.37
  Top 0.406: R8.1 88.81,43.41 89.6,44.2 U2.3 92.97,44.2 93.98,43.18 93.98,40.64 | U6.7 114.56,60.07 114.94,59.69 114.94,54.61 114.3,53.98 v113.03,53.98 111.76,53.98 110.75,52.96 R29.2 105.7,51.09 102.23,47.62 102.23,42.55 100.33,40.64 93.98,40.64 | 93.98,40.64 89.53,40.64 88.27,39.37
  Bottom 0.406: SV2.2 113.28,53.72 v113.03,53.98
TEMP1/SCL1  (via drill 0.51)
  Top 0.406: J4.5 72.77,56.26 71.12,54.61 v71.12,53.98 | v74.3,48.9 74.93,48.9 76.2,47.62 76.2,46.99 77.72,45.47 U1.7 82.54,45.47 R7.2 R13.2
  Bottom 0.406: v71.12,53.98 71.12,52.07 v74.3,48.9
TEMP2/SCL2  (via drill 0.51)
  Top 0.406: J5.5 89.28,56.26 87.63,54.61 v87.63,53.98 | R14.2 R9.2 99.05,45.47 U2.7 94.23,45.47 93.28,46.42 93.28,46.93 91.95,48.26 v91.44,48.26
  Bottom 0.406: v87.63,53.98 87.63,52.07 v91.44,48.26
TEMP3/SCL3  (via drill 0.51)
  Top 0.406: J6.5 56.26,56.26 54.61,54.61 v54.61,53.98 | v57.78,48.9 58.42,48.9 59.69,47.62 59.69,46.99 61.22,45.47 U3.7 66.03,45.47 R11.2 R15.2
  Bottom 0.406: v54.61,53.98 54.61,52.07 v57.78,48.9
USB+
  Top 0.254: U7.36 82.7,16.02 81.92,15.24 81.92,14.61
  Top 0.406: J7.D- 6.75,10.55 6.99,10.79 7.62,10.79
  Top 1.016: 9.53,10.79 10.79,10.79
  Top 1.067: 7.62,10.79 9.53,10.79 | 10.79,10.79 15.24,6.35 80.64,6.35 81.92,7.62 81.92,14.61
USB-
  Top 0.254: U7.37 83.2,14.62 83.19,14.61
  Top 0.406: J7.D+ 6.61,9.9 6.99,9.53 7.62,9.53
  Top 1.016: 9.53,9.53 10.16,9.53
  Top 1.067: 7.62,9.53 9.53,9.53 | 10.16,9.53 14.61,5.08 81.28,5.08 83.19,6.99 83.19,14.61
USBID  (via drill 0.51)
  Top 0.254: v78.74,17.78 78.96,18 79.44,18 79.53,18.1 81.1,18.1 U7.33
  Top 0.406: R37.1 9.53,4.57 9.53,6.35 8.89,6.99 6.99,6.99 6.35,7.62 6.35,8.89 5.99,9.26 J7.ID 3.76,9.26 3.49,9.53 3.49,11.75 3.81,12.06 5.71,12.06 7.62,13.97 19.68,13.97 20,13.65 20,11.11 21.59,9.53 72.39,9.53 v76.2,13.34
  Bottom 0.254: v78.74,17.78 78.11,17.14 78.11,15.24 v76.2,13.34
V+
  Top 1.27: K2.7 12.26,27.57 K1.1 13.18,27.78 20.32,34.92 20.32,38.13 F1.2
VBUS  (via drill 0.51)
  Top 0.254: U7.34 81.7,17.25 81.44,16.99 80.33,16.99 v80.01,17.3
  Top 0.406: J7.VBUS 6.12,11.21 7.62,12.7 13.34,12.7 17.14,8.89 73.66,8.89 v77.47,12.7 | 18.66,12.7 F3.1
  Top 1.016: 18.66,12.7 13.34,12.7
  Bottom 0.254: v80.01,17.3 79.53,17.3 78.8,16.57 78.8,15.24 77.47,13.91 v77.47,12.7
(copper drawn outside any net)
  shapes: Top circle x2

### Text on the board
tNames: 2A time lag | ANEMOMETER | SENSOR A | SENSOR B | SENSOR C | 0,5A | I2C_A | V- | Vin+ | SDA | SCL | Vin- | V+ | I2C_B | V- | Vin+ | Out1+ | Vin- | Out1+ | Out1- | SDA | Out1- | Out2+ | Out2- | SCL | MCLR | VCC | GND | V+ | Out2+ | PIN38/PGD | PIN37/PGC | I2C_C | V- | Out2- | SDA | SCL | V+ | MCLR | WATCHDOG RESET | BOOT | GND | Thomas H-TNA Software R3A-2014
bNames: Thomas H-TNA Software R2A-2013

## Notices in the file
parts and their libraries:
SparkFun: Licensing: CC v3.0 Share-Alike You are welcome to use this library for commercial purposes.
SparkFun-Aesthetics: Released under the Creative Commons Attribution Share-Alike 3.0 License
SparkFun-Aesthetics: http://creativecommons.org/licenses/by-sa/3.0
